(* Logix 5000 AddOnInstructionDefinition export Banner_TLF100_Param_v4; software revision 33.00 *)

TYPE Banner_IOL_Port_v4 :   // UDT that has all of the data items necessary to communicate with a specific Port on a IO-Link Master
STRUCT
   Port_Controlled : INT;   // Each bit represents a port on an IO-Link Master. Set to 1 to tell AOI to control that port.
   Port_Activate : INT;   // Each bit represents a port on an IO-Link Master. When ON that port will process any commands in queue.
   Port_Read : INT;   // Each bit represents a port on an IO-Link Master. Used to determine when device AOI has requested a Read command.
   Port_Write : INT;   // Each bit represents a port on an IO-Link Master. Used to determine when device AOI has requested a Write command.
   Port_RW_Complete : INT;   // Each bit represents a port on an IO-Link Master. Tells device AOI that Read or Write request has been completed.
   Port_Device_Read : INT;
   Data_Transfer : SINT[190];   // Array to transfer data from IO-Master to device AOIs.
END_STRUCT
END_TYPE

TYPE Banner_TLF100_General_Level_Config_v4 :
STRUCT
   BG_Color : SINT;   // Background Color. 0 = Green, 1 = Red, 2 = Orange, 3 = Amber, 4 = Yellow, 5 = Lime Green, 6 = Spring Green, 7 = Cyan, 8 = Sky Blue, 9 = Blue, 10 = Violet, 11 = Magenta, 12 = Rose, 13 = White, 14 = Custom, 15 = Custom 2.
   BG_Intensity : SINT;   // 0 = High, 1 = Low, 2 = Medium, 3 = Off, 4 = Custom
   Dominance : SINT;   // 0 = Non-Dominant, 1 = Dominant
   Sub_Segment_Style : SINT;   // 0 = Solid, 1 = Analog
   Filtering : SINT;   // 0 = None, 1 = Low, 2 = Medium, 3 = High
   Hysteresis : SINT;   // 0 = None, 1 = Low, 2 = Medium, 3 = High
   Full_Scale_Value : INT;   // Default value is 100
END_STRUCT
END_TYPE

TYPE Banner_TLF100_General_Seg_Config_v4 :
STRUCT
   Segment_Mode : INT;   // 0 = Manual Segment Config, 1 = 1 Segment, 2 = 2 Segments, 3 = 3 Segments, 4 = 4 Segments
   Background_Color : INT;   // 0 = Green, 1 = Red, 2 = Orange, 3 = Amber, 4 = Yellow, 5 = Lime Green, 6 = Spring Green, 7 = Cyan, 8 = Sky Blue, 9 = Blue, 10 = Violet, 11 = Magenta, 12 = Rose, 13 = White, 14 = Custom, 15 = Custom 2
   Background_Intensity : SINT;   // 0 = High, 1 = Low, 2 = Medium, 3 = Off, 4 = Custom
   Animation_Synchro : SINT;   // 0 = Animation Sync Disabled, 1 = Animation Sync Enabled
END_STRUCT
END_TYPE

TYPE Banner_TLF100_Level_Base_Config_v4 :
STRUCT
   Animation : INT;   // 0 = Off, 1 = Steady, 2 = Flash, 3 = Two Color Flash, 4 = Two Color Shift, 5 = Scroll, 6 = Center Scroll, 7 = Bounce, 8 = Center Bounce, 9 = Intensity Sweep, 10 = Two Color Sweep, 11 = Spectrum, 12 = Single End Steady, 13 = Daylight White, 14 = Custom 1, 15 = Custom 2
   Color_1 : INT;   // 0 = Green, 1 = Red, 2 = Orange, 3 = Amber, 4 = Yellow, 5 = Lime Green, 6 = Spring Green, 7 = Cyan, 8 = Sky Blue, 9 = Blue, 10 = Violet, 11 = Magenta, 12 = Rose, 13 = White, 14 = Custom, 15 = Custom 2
   Color_1_Intensity : SINT;   // 0 = High, 1 = Low, 2 = Medium, 3 = Off, 4 = Custom
   Speed : SINT;   // 0 = Medium, 1 = Fast, 2 = Slow, 3 = Custom Flash Rate
   Pulse_Pattern : SINT;   // 0 = Normal, 1 = Strobe, 2 = Three Pulse, 3 = SOS, 4 = Random
   Color_2 : INT;   // 0 = Green, 1 = Red, 2 = Orange, 3 = Amber, 4 = Yellow, 5 = Lime Green, 6 = Spring Green, 7 = Cyan, 8 = Sky Blue, 9 = Blue, 10 = Violet, 11 = Magenta, 12 = Rose, 13 = White, 14 = Custom, 15 = Custom 2
   Color_2_Intensity : INT;   // 0 = High, 1 = Low, 2 = Medium, 3 = Off, 4 = Custom
   Scroll_Bounce_Style : SINT;   // 0 = Solid, 1 = Tail, 2 = Ripple
   Percent_Width_of_Color_1 : SINT;   // 0 to 100. The size of the scrolling segement
   Direction : SINT;   // 0 = Up, 1 = Down
   Audible : SINT;   // 0 = Pulse, 1 = Wobble, 2 = Strobe, 4 = Whoop, 5 = Stacatto, 6 = Siren, 8 = Continuous 1, 9 = Continuous 2, 16 = Jingle, 17 = Melody 1, 18 = Melody 2, 19 = Melody 3, 20 = Custom
   Audible_Volume : SINT;   // 0 = Off, 1 = Low, 2 = Medium, 3 = High
END_STRUCT
END_TYPE

TYPE Banner_TLF100_RD_v4 :   // UDT that stores the Read Data for a TLF100 Pro.
STRUCT
   Master_Cycle_Time : INT;
   Min_Cycle_Time : INT;
   M_Sequence_Capability : INT;
   IO_Link_Version_ID : INT;
   Process_Data_Input_Length : INT;
   Process_Data_Output_Length : INT;
   Combined_Vendor_ID : DINT;   // IO-Link Vendor ID
   Vendor_ID1 : INT;
   Vendor_ID2 : INT;
   Combined_Device_ID : DINT;   // IO-Link Device ID
   Device_ID1 : INT;
   Device_ID2 : INT;
   Device_ID3 : INT;
   Serial_Number : STRING;
END_STRUCT
END_TYPE

TYPE Banner_TLF100_SegConfig_v4 :   // Basic parameters for a TLF100 segment.
STRUCT
   Animation : SINT;   // 0 = Off, 1 = Steady, 2 = Flash, 3 = Two Color, 4 = Half/Half, 5 = Half/Half Rotate, 6 = Chase, 7 = Intesnity Sweep
   Color_1 : INT;   // 0 = Green, 1 = Red, 2 = Orange, 3 = Amber, 4 = Yellow, 5 = Lime Green, 6 = Spring Green, 7 = Cyan, 8 = Sky Blue, 9 = Blue, 10 = Violet, 11 = Magenta, 12 = Rose, 13 = White, 14 = Custom, 15 = Custom 2
   Color_1_Intensity : SINT;   // 0 = High, 1 = Low, 2 = Medium, 3 = Off, 4 = Custom
   Speed : SINT;   // 0 = Medium, 1 = Fast, 2 = Slow, 3 = Custom
   Pulse_Pattern : SINT;   // 0 = Normal, 1 = Strobe, 2 = Three Pulse, 3 = SOS, 4 = Random
   Color_2 : SINT;   // 0 = Green, 1 = Red, 2 = Orange, 3 = Amber, 4 = Yellow, 5 = Lime Green, 6 = Spring Green, 7 = Cyan, 8 = Sky Blue, 9 = Blue, 10 = Violet, 11 = Magenta, 12 = Rose, 13 = White, 14 = Custom, 15 = Custom 2
   Color_2_Intensity : SINT;   // 0 = High, 1 = Low, 2 = Medium, 3 = Off, 4 = Custom
   Scroll_Bounce : SINT;   // 0 = Solid, 1 = Tail, 2 = Ripple
   Percent_Width_of_C1 : SINT;   // 1 to 100 percent
   Direction : SINT;   // 0 = Up, 1 = Down
END_STRUCT
END_TYPE

TYPE Banner_TLF100_Threshold_Config_v4 :
STRUCT
   Threshold_Enable : SINT;   // 0 = Threshold Disabled, 1 = Threshold Enabled
   Threshold_Value_Percent : SINT;   // 0 to 100 percent.
   Threshold_Comparison : SINT;   // 0 = Less than or equal to, 1 = Greater than or equal to
   Threshold_Override : SINT;   // 0 = Override not enabled, 1 = Override Enabled
   Animation : INT;   // 0 = Off, 1 = Steady, 2 = Flash, 3 = Two Color Flash, 4 = Two Color Shift, 5 = Scroll, 6 = Center Scroll, 7 = Bounce, 8 = Center Bounce, 9 = Intensity Sweep, 10 = Two Color Sweep, 11 = Spectrum, 12 = Single End Steady, 13 = Single End Flash
   Color_1 : INT;   // 0 = Green, 1 = Red, 2 = Orange, 3 = Amber, 4 = Yellow, 5 = Lime Green, 6 = Spring Green, 7 = Cyan, 8 = Sky Blue, 9 = Blue, 10 = Violet, 11 = Magenta, 12 = Rose, 13 = White, 14 = Custom, 15 = Custom 2
   Color_1_Intensity : SINT;   // 0 = High, 1 = Low, 2 = Medium, 3 = Off, 4 = Custom
   Speed : SINT;   // 0 = Medium, 1 = Fast, 2 = Slow, 3 = Custom Flash Rate
   Pulse_Pattern : SINT;   // 0 = Normal, 1 = Strobe, 2 = Three Pulse, 3 = SOS, 4 = Random
   Color_2 : INT;   // 0 = Green, 1 = Red, 2 = Orange, 3 = Amber, 4 = Yellow, 5 = Lime Green, 6 = Spring Green, 7 = Cyan, 8 = Sky Blue, 9 = Blue, 10 = Violet, 11 = Magenta, 12 = Rose, 13 = White, 14 = Custom, 15 = Custom 2
   Color_2_Intensity : SINT;   // 0 = High, 1 = Low, 2 = Medium, 3 = Off, 4 = Custom
   Scroll_Bounce_Style : SINT;   // 0 = Solid, 1 = Tail, 2 = Ripple
   Percent_Width_of_Color_1 : SINT;   // 0 to 100
   Direction : SINT;   // 0 = Up, 1 = Down
   Audible_Type : SINT;   // 0 = Pulse, 1 = Wobble, 2 = Strobe, 4 = Whoop, 5 = Stacatto, 6 = Siren, 8 = Continuous 1, 9 = Continuous 2, 12 = Sync, 16 = Jingle, 17 = Melody 1, 18 = Melody 2, 19 = Melody 3, 20 = Custom
   Audible_Volume : SINT;   // 0 = Off, 1 = Low, 2 = Medium, 3 = High
END_STRUCT
END_TYPE

TYPE Banner_TLF100_v4 :   // All of the parameters for a TLF100.
STRUCT
   Initial_Global_Read : BOOL;   // Determines if all of the IO-Link data has been read into the PLC yet
   Command : INT;   // Value placed in here will activate a read or write to a specifc IO-Link Index
   Read : Banner_TLF100_RD_v4;   // Read Only Data
   Write : Banner_TLF100_WD_v4;   // Write Data
   Archive : Banner_TLF100_WD_v4;   // Archive of the Write Data
   Reset : BOOL;   // Resets AOI. This will force a complete parameter read of the sensor.
END_STRUCT
END_TYPE

TYPE Banner_TLF100_WD_v4 :   // UDT that stores the Write Data for a TLF100.
STRUCT
   System_Command : INT;   // See IODD file for list of commands that can be activated via the System Command interface
   Parameter_Access_Lock : SINT;   // Write access to all parameters is prohibited while value is 1. Only this parameter can be adjusted when value is 1.
   Data_Storage_Lock : SINT;   // Automatic data storage is disabled when this value is equal to 1. Read access is not affected.
   Local_Parameterization_Lock : SINT;   // Parameterization via local control elements on device is disabled.
   Local_User_Interface_Lock : SINT;   // Operation of local user interface is disabled.
   Operating_Mode_Selection : SINT;   // 0 = Segment Mode, 1 = Run Mode, 2= Level Mode, 3 = Adv Seg Mode, 4 = Demo Mode
   General_Segment_Config : Banner_TLF100_General_Seg_Config_v4;
   Segment_Config : Banner_TLF100_SegConfig_v4[5];
   General_Level_Config : Banner_TLF100_General_Level_Config_v4;
   Level_Base_Config : Banner_TLF100_Level_Base_Config_v4;
   Level_Threshold_Config : Banner_TLF100_Threshold_Config_v4[5];
   Custom_1_Red : INT;   // 0 to 255. Value of the Red portion of the RGB color value for Custom 1
   Custom_1_Green : INT;   // 0 to 255. Value of the Green portion of the RGB color value for Custom 1.
   Custom_1_Blue : INT;   // 0 to 255. Value of the Blue portion of the RGB color value for Custom 1.
   Custom_2_Red : INT;   // 0 to 255. Value of the Red portion of the RGB color value for Custom 2.
   Custom_2_Green : INT;   // 0 to 255. Value of the Green portion of the RGB color value for Custom 2.
   Custom_2_Blue : INT;   // 0 to 255. Value of the Blue portion of the RGB color value for Custom 2.
   Orientation : SINT;   // 0 = Standard, 1 = Inverted
   Custom_Intensity : SINT;   // 0 to 100
   Custom_Frequency : INT;   // 0 to 255
   Audible : SINT;   // 0 = Pulse, 1 = Wobble, 2 = Strobe, 4 = Whoop, 5 = Stacatto, 6 = Siren, 8 = Continuous 1, 9 = Continuous 2, 16 = Jingle, 17 = Melody 1, 18 = Melody 2, 19 = Melody 3, 20 = Custom
   Audible_Volume : SINT;   // 0 = Off, 1 = Low, 2 = Medium, 3 = High
   Custom_Type : SINT;   // 0 = Beep, 1 = Sweep, 2 = Tone
   Custom_Sweep_Type : SINT;   // 0 = Up, 1 = Down, 2 = Up Down, 3 = Down Up
   Custom_Freq_1 : SINT;   // 0 = Off, 1 = Low, 2 = Standard, 3 = High
   Custom_Freq_2 : SINT;   // 0 = Off, 1 = Low, 2 = Standard, 3 = High
END_STRUCT
END_TYPE

ADD_ON_INSTRUCTION Banner_TLF100_Param_v4   (* revision 4.1, vendor Banner Engineering *)
// AOI to read and write parameter data to an IO-Link TLF100.
VAR_IN_OUT
   TLF100 : Banner_TLF100_v4; {required}
   Port_Data : Banner_IOL_Port_v4; {required}
END_VAR
VAR_INPUT
   Port : INT; {required}   // Port Number that device is plugged into.
END_VAR
VAR
   Local_Control : DINT; {access None}
   Global_Read_Command_Value : INT; {access None}
   Global_Write_Command_Value : INT; {access None}
   Command_Being_Processed : BOOL; {access None}
   Update_Archive : BOOL; {access None}
   Index_Write_Inprocess : DINT; {access None}
   Index_Write_Control : DINT; {access None}
   Inprocess_Index : DINT; {access None}
   Index_R : DINT; {access None}
   BS_Index : DINT; {access None}
   Index_W : DINT; {access None}
   W_Index : DINT; {access None}
   Index_Segment_Read : DINT; {access None}
   GT_Index2 : DINT; {access None}
   GT_Index1 : DINT; {access None}
   LT_Index2 : DINT; {access None}
   LT_Index1 : DINT; {access None}
END_VAR

ROUTINE Logic   (* ladder *)
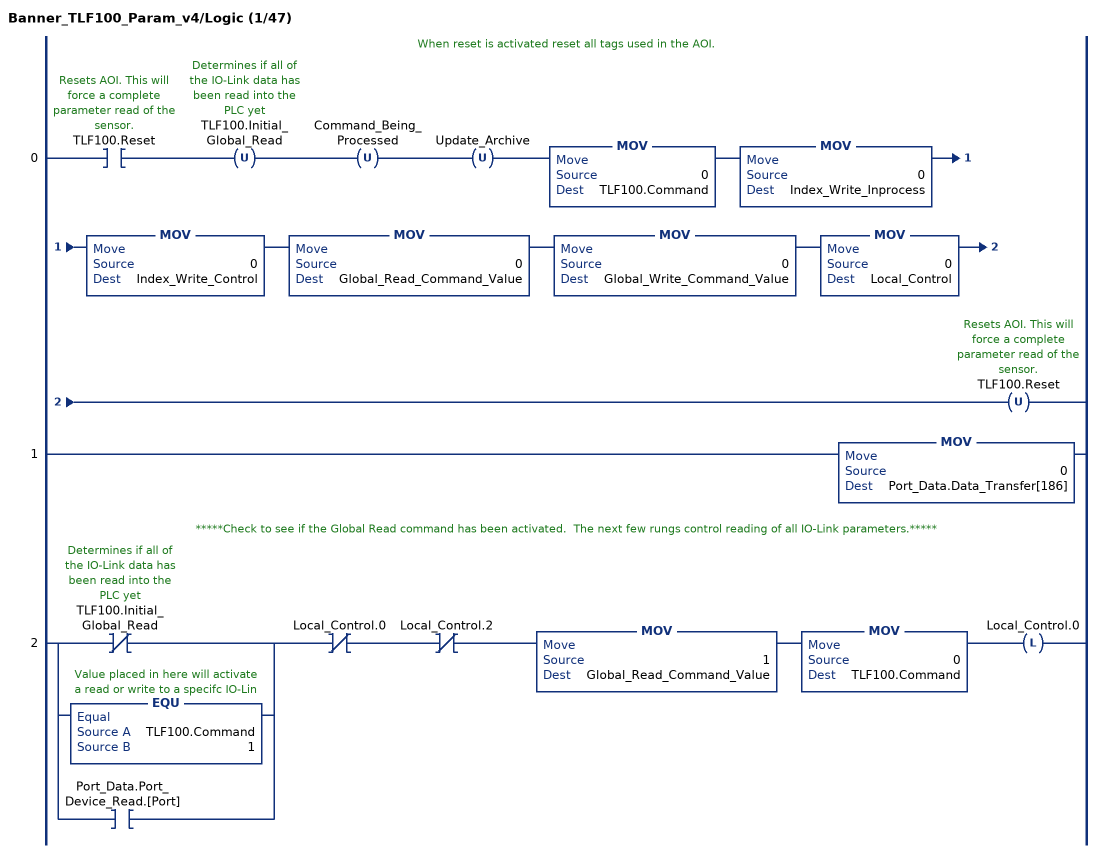
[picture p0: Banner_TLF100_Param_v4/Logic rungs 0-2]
   // When reset is activated reset all tags used in the AOI.
   0: XIC(TLF100.Reset)OTU(TLF100.Initial_Global_Read)OTU(Command_Being_Processed)OTU(Update_Archive)MOV(0,TLF100.Command)MOV(0,Index_Write_Inprocess)MOV(0,Index_Write_Control)MOV(0,Global_Read_Command_Value)MOV(0,Global_Write_Command_Value)MOV(0,Local_Control)OTU(TLF100.Reset);
   1: MOV(0,Port_Data.Data_Transfer[186]);
   // *****Check to see if the Global Read command has been activated.  The next few rungs control reading of all IO-Link parameters.*****
   2: [XIO(TLF100.Initial_Global_Read) ,EQU(TLF100.Command,1) ,XIC(Port_Data.Port_Device_Read.[Port]) ]XIO(Local_Control.0)XIO(Local_Control.2)MOV(1,Global_Read_Command_Value)MOV(0,TLF100.Command)OTL(Local_Control.0);
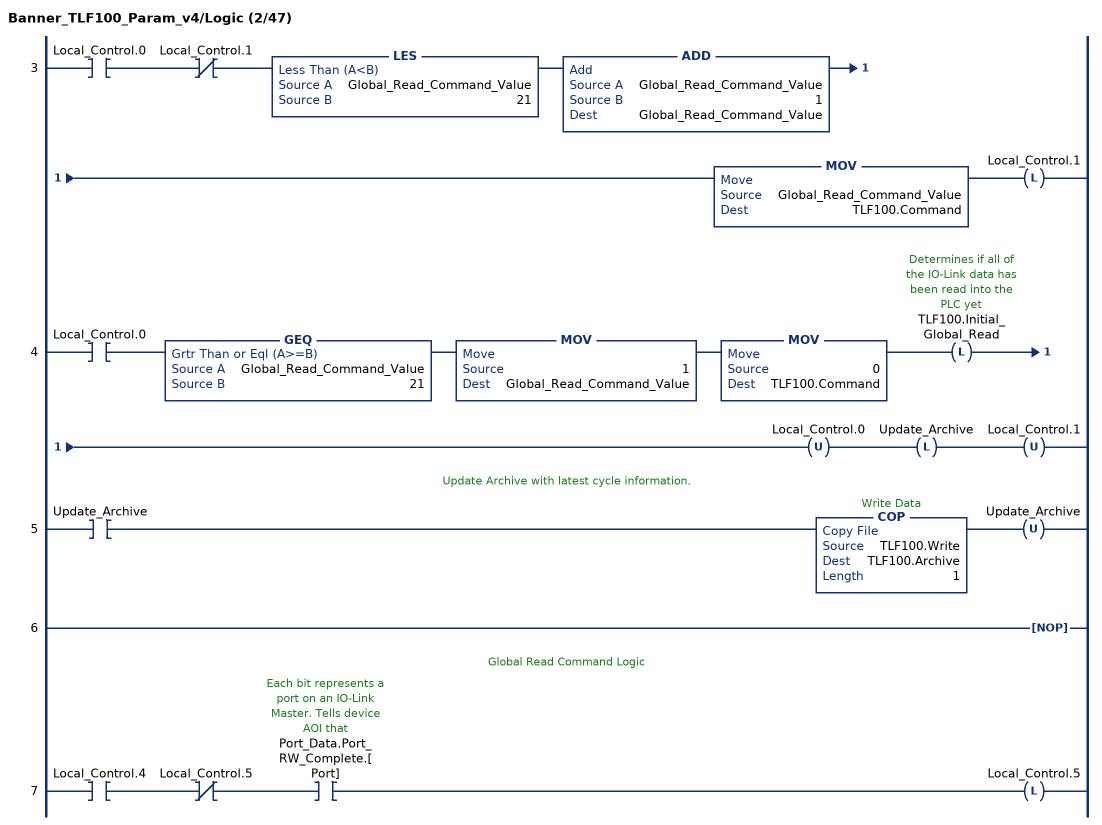
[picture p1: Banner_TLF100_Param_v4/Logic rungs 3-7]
   3: XIC(Local_Control.0)XIO(Local_Control.1)LES(Global_Read_Command_Value,21)ADD(Global_Read_Command_Value,1,Global_Read_Command_Value)MOV(Global_Read_Command_Value,TLF100.Command)OTL(Local_Control.1);
   4: XIC(Local_Control.0)GEQ(Global_Read_Command_Value,21)MOV(1,Global_Read_Command_Value)MOV(0,TLF100.Command)OTL(TLF100.Initial_Global_Read)OTU(Local_Control.0)OTL(Update_Archive)OTU(Local_Control.1);
   // Update Archive with latest cycle information.
   5: XIC(Update_Archive)COP(TLF100.Write,TLF100.Archive,1)OTU(Update_Archive);
   6: NOP();
   // Global Read Command Logic
   7: XIC(Local_Control.4)XIO(Local_Control.5)XIC(Port_Data.Port_RW_Complete.[Port])OTL(Local_Control.5);
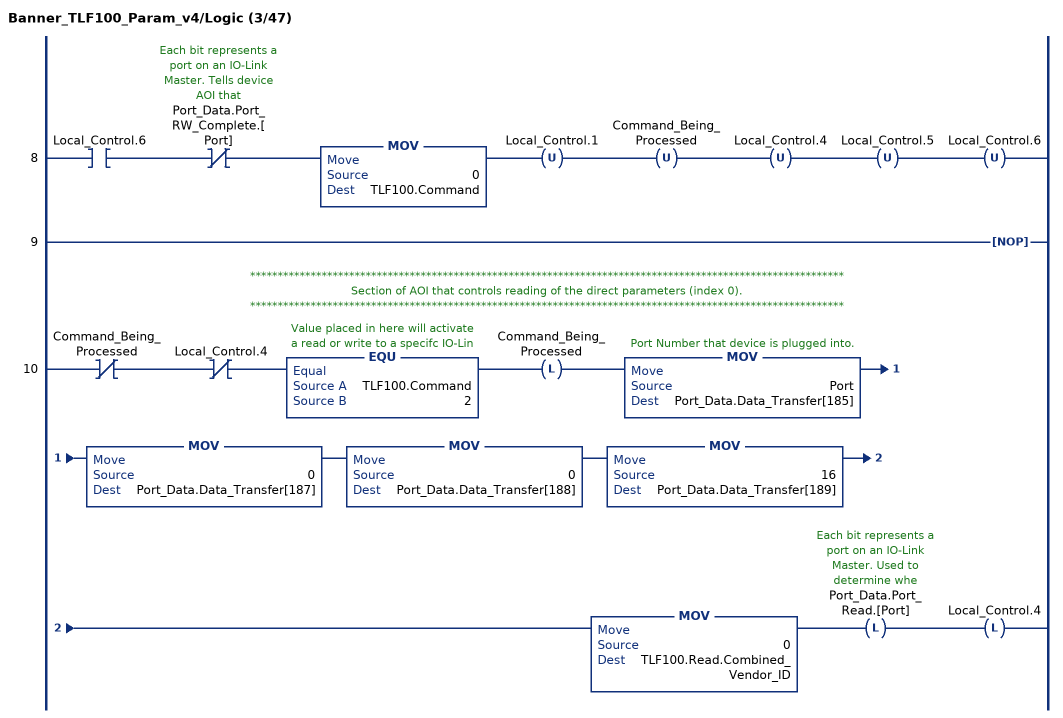
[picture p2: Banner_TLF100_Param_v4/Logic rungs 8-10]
   8: XIC(Local_Control.6)XIO(Port_Data.Port_RW_Complete.[Port])MOV(0,TLF100.Command)OTU(Local_Control.1)OTU(Command_Being_Processed)OTU(Local_Control.4)OTU(Local_Control.5)OTU(Local_Control.6);
   9: NOP();
   // ************************************************************************************************************
   // Section of AOI that controls reading of the direct parameters (index 0).
   // ************************************************************************************************************
   10: XIO(Command_Being_Processed)XIO(Local_Control.4)EQU(TLF100.Command,2)OTL(Command_Being_Processed)MOV(Port,Port_Data.Data_Transfer[185])MOV(0,Port_Data.Data_Transfer[187])MOV(0,Port_Data.Data_Transfer[188])MOV(16,Port_Data.Data_Transfer[189])MOV(0,TLF100.Read.Combined_Vendor_ID)OTL(Port_Data.Port_Read.[Port])OTL(Local_Control.4);
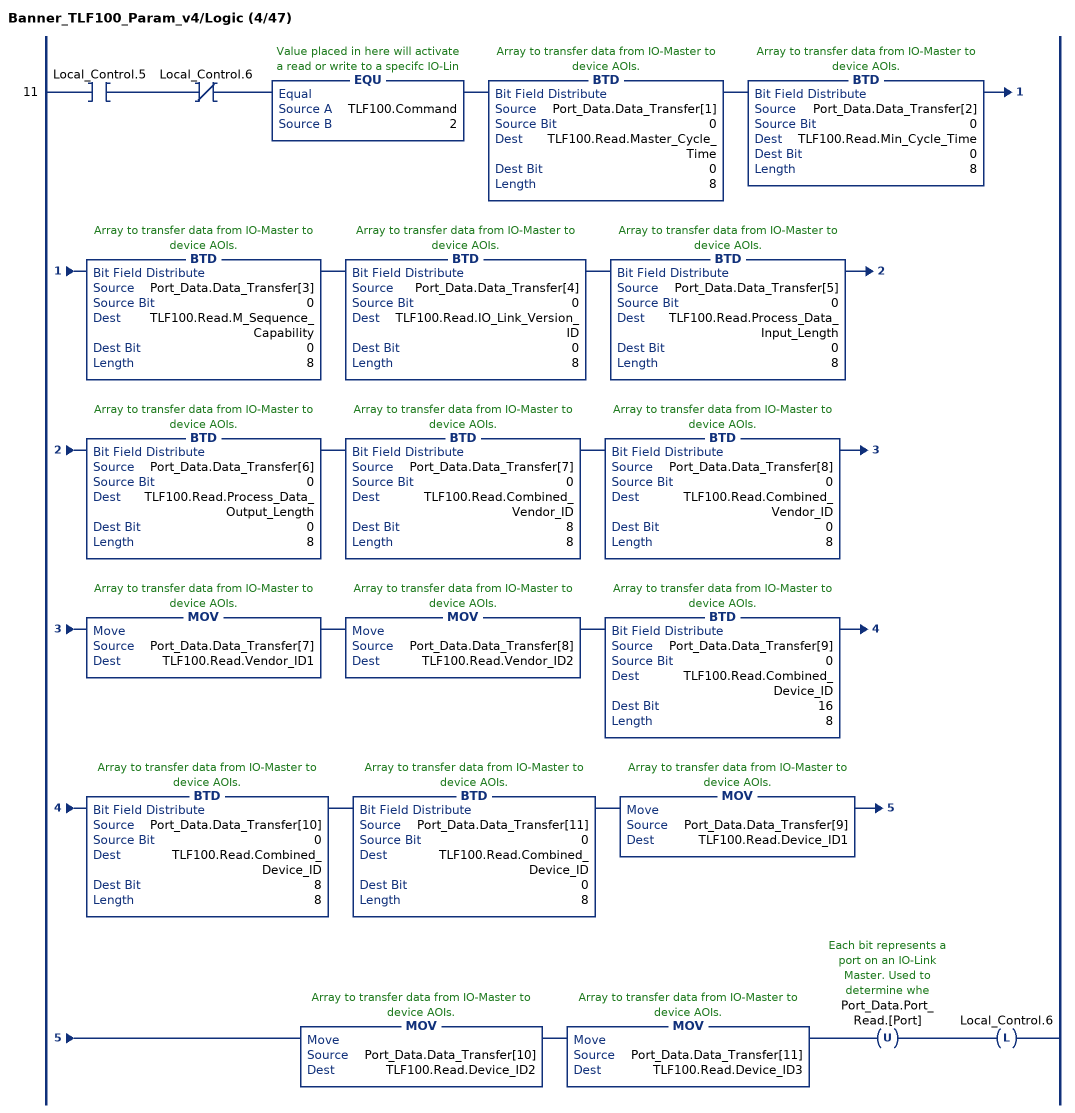
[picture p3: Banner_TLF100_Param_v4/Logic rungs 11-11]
   11: XIC(Local_Control.5)XIO(Local_Control.6)EQU(TLF100.Command,2)BTD(Port_Data.Data_Transfer[1],0,TLF100.Read.Master_Cycle_Time,0,8)BTD(Port_Data.Data_Transfer[2],0,TLF100.Read.Min_Cycle_Time,0,8)BTD(Port_Data.Data_Transfer[3],0,TLF100.Read.M_Sequence_Capability,0,8)BTD(Port_Data.Data_Transfer[4],0,TLF100.Read.IO_Link_Version_ID,0,8)BTD(Port_Data.Data_Transfer[5],0,TLF100.Read.Process_Data_Input_Length,0,8)BTD(Port_Data.Data_Transfer[6],0,TLF100.Read.Process_Data_Output_Length,0,8)BTD(Port_Data.Data_Transfer[7],0,TLF100.Read.Combined_Vendor_ID,8,8)BTD(Port_Data.Data_Transfer[8],0,TLF100.Read.Combined_Vendor_ID,0,8)MOV(Port_Data.Data_Transfer[7],TLF100.Read.Vendor_ID1)MOV(Port_Data.Data_Transfer[8],TLF100.Read.Vendor_ID2)BTD(Port_Data.Data_Transfer[9],0,TLF100.Read.Combined_Device_ID,16,8)BTD(Port_Data.Data_Transfer[10],0,TLF100.Read.Combined_Device_ID,8,8)BTD(Port_Data.Data_Transfer[11],0,TLF100.Read.Combined_Device_ID,0,8)MOV(Port_Data.Data_Transfer[9],TLF100.Read.Device_ID1)MOV(Port_Data.Data_Transfer[10],TLF100.Read.Device_ID2)MOV(Port_Data.Data_Transfer[11],TLF100.Read.Device_ID3)OTU(Port_Data.Port_Read.[Port])OTL(Local_Control.6);
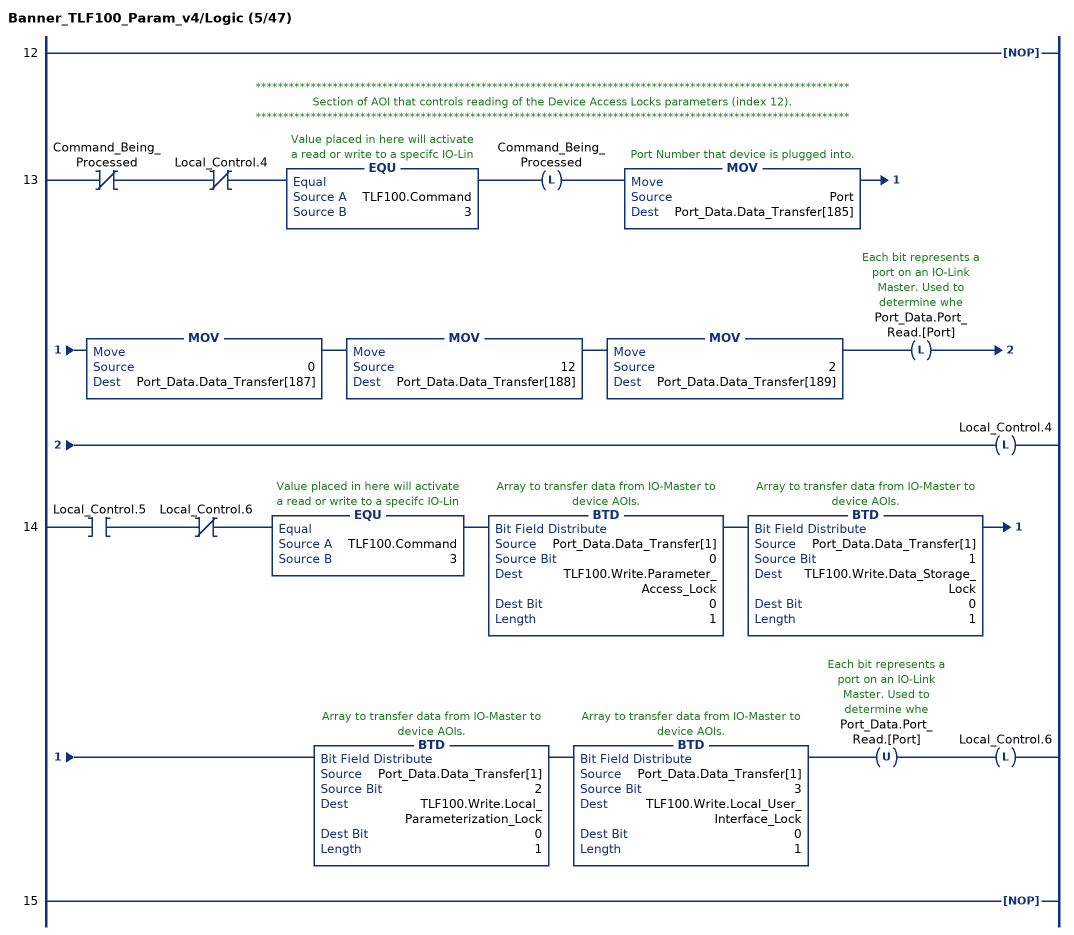
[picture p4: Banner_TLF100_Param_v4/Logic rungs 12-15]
   12: NOP();
   // ************************************************************************************************************
   // Section of AOI that controls reading of the Device Access Locks parameters (index 12).
   // ************************************************************************************************************
   13: XIO(Command_Being_Processed)XIO(Local_Control.4)EQU(TLF100.Command,3)OTL(Command_Being_Processed)MOV(Port,Port_Data.Data_Transfer[185])MOV(0,Port_Data.Data_Transfer[187])MOV(12,Port_Data.Data_Transfer[188])MOV(2,Port_Data.Data_Transfer[189])OTL(Port_Data.Port_Read.[Port])OTL(Local_Control.4);
   14: XIC(Local_Control.5)XIO(Local_Control.6)EQU(TLF100.Command,3)BTD(Port_Data.Data_Transfer[1],0,TLF100.Write.Parameter_Access_Lock,0,1)BTD(Port_Data.Data_Transfer[1],1,TLF100.Write.Data_Storage_Lock,0,1)BTD(Port_Data.Data_Transfer[1],2,TLF100.Write.Local_Parameterization_Lock,0,1)BTD(Port_Data.Data_Transfer[1],3,TLF100.Write.Local_User_Interface_Lock,0,1)OTU(Port_Data.Port_Read.[Port])OTL(Local_Control.6);
   15: NOP();
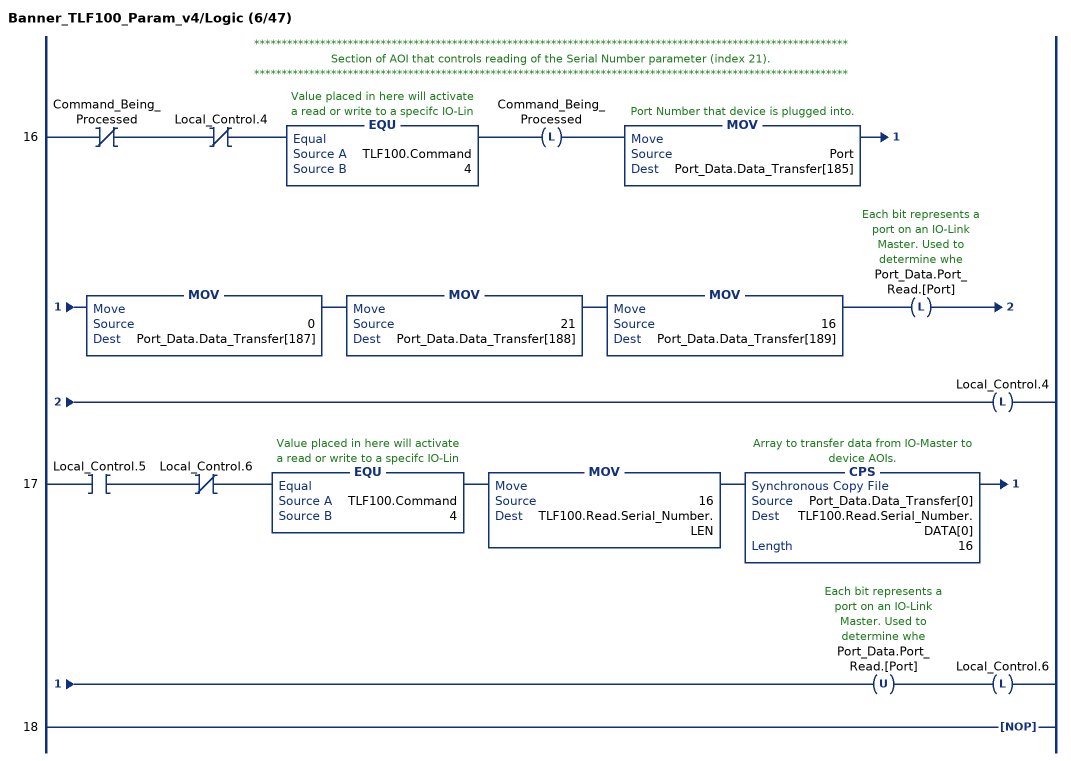
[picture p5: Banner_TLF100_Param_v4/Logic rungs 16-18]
   // ************************************************************************************************************
   // Section of AOI that controls reading of the Serial Number parameter (index 21).
   // ************************************************************************************************************
   16: XIO(Command_Being_Processed)XIO(Local_Control.4)EQU(TLF100.Command,4)OTL(Command_Being_Processed)MOV(Port,Port_Data.Data_Transfer[185])MOV(0,Port_Data.Data_Transfer[187])MOV(21,Port_Data.Data_Transfer[188])MOV(16,Port_Data.Data_Transfer[189])OTL(Port_Data.Port_Read.[Port])OTL(Local_Control.4);
   17: XIC(Local_Control.5)XIO(Local_Control.6)EQU(TLF100.Command,4)MOV(16,TLF100.Read.Serial_Number.LEN)CPS(Port_Data.Data_Transfer[0],TLF100.Read.Serial_Number.DATA[0],16)OTU(Port_Data.Port_Read.[Port])OTL(Local_Control.6);
   18: NOP();
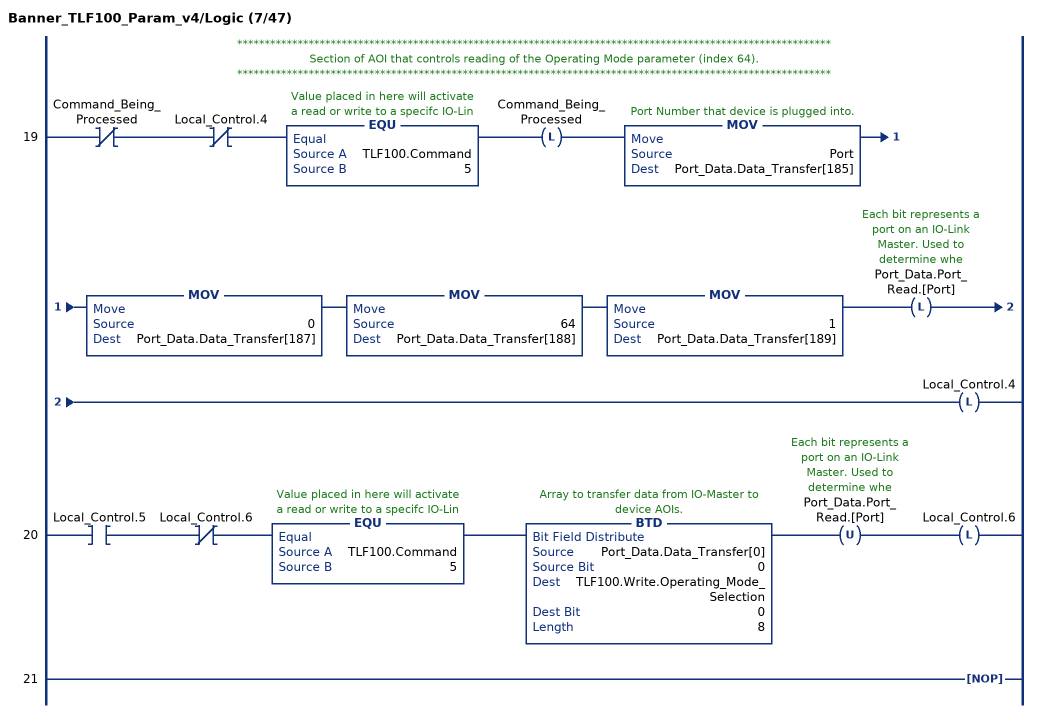
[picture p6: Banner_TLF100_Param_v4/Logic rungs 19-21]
   // ************************************************************************************************************
   // Section of AOI that controls reading of the Operating Mode parameter (index 64).
   // ************************************************************************************************************
   19: XIO(Command_Being_Processed)XIO(Local_Control.4)EQU(TLF100.Command,5)OTL(Command_Being_Processed)MOV(Port,Port_Data.Data_Transfer[185])MOV(0,Port_Data.Data_Transfer[187])MOV(64,Port_Data.Data_Transfer[188])MOV(1,Port_Data.Data_Transfer[189])OTL(Port_Data.Port_Read.[Port])OTL(Local_Control.4);
   20: XIC(Local_Control.5)XIO(Local_Control.6)EQU(TLF100.Command,5)BTD(Port_Data.Data_Transfer[0],0,TLF100.Write.Operating_Mode_Selection,0,8)OTU(Port_Data.Port_Read.[Port])OTL(Local_Control.6);
   21: NOP();
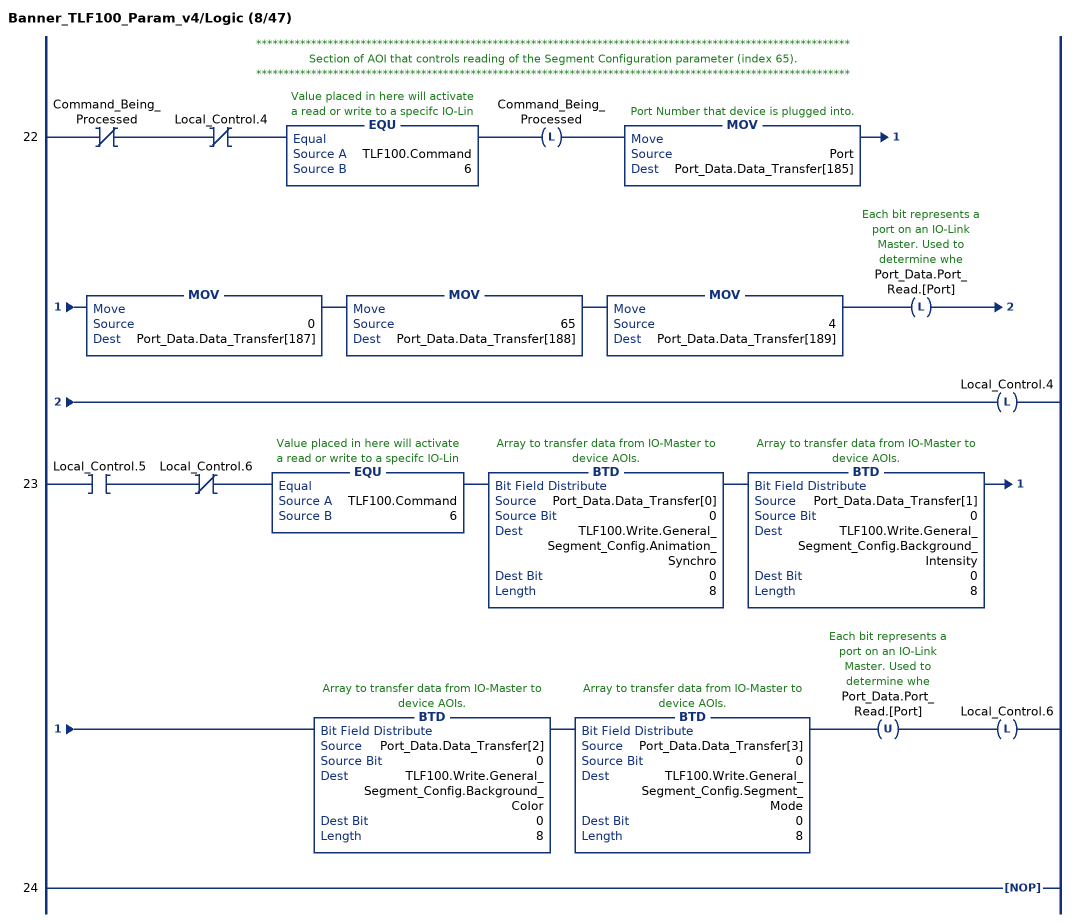
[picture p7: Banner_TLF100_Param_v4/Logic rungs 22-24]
   // ************************************************************************************************************
   // Section of AOI that controls reading of the Segment Configuration parameter (index 65).
   // ************************************************************************************************************
   22: XIO(Command_Being_Processed)XIO(Local_Control.4)EQU(TLF100.Command,6)OTL(Command_Being_Processed)MOV(Port,Port_Data.Data_Transfer[185])MOV(0,Port_Data.Data_Transfer[187])MOV(65,Port_Data.Data_Transfer[188])MOV(4,Port_Data.Data_Transfer[189])OTL(Port_Data.Port_Read.[Port])OTL(Local_Control.4);
   23: XIC(Local_Control.5)XIO(Local_Control.6)EQU(TLF100.Command,6)BTD(Port_Data.Data_Transfer[0],0,TLF100.Write.General_Segment_Config.Animation_Synchro,0,8)BTD(Port_Data.Data_Transfer[1],0,TLF100.Write.General_Segment_Config.Background_Intensity,0,8)BTD(Port_Data.Data_Transfer[2],0,TLF100.Write.General_Segment_Config.Background_Color,0,8)BTD(Port_Data.Data_Transfer[3],0,TLF100.Write.General_Segment_Config.Segment_Mode,0,8)OTU(Port_Data.Port_Read.[Port])OTL(Local_Control.6);
   24: NOP();
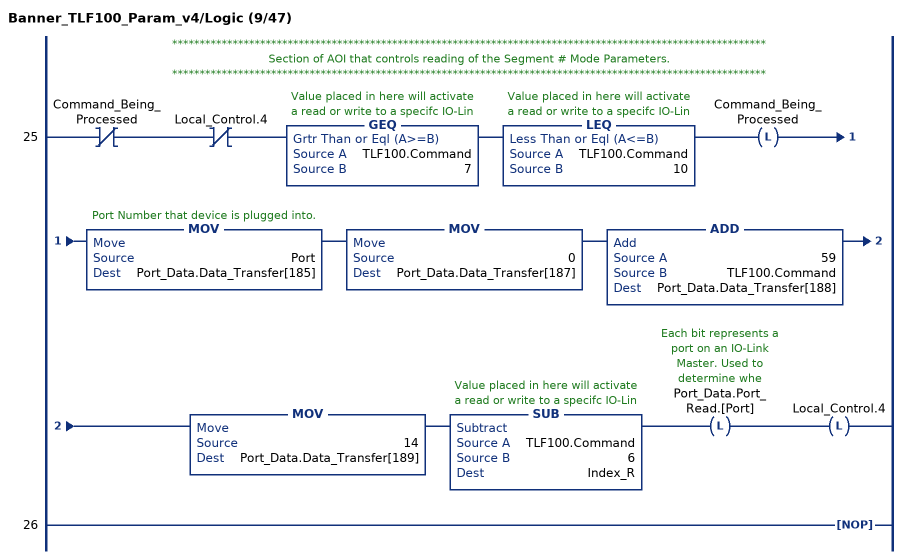
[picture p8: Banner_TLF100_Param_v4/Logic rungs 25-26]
   // ************************************************************************************************************
   // Section of AOI that controls reading of the Segment # Mode Parameters.
   // ************************************************************************************************************
   25: XIO(Command_Being_Processed)XIO(Local_Control.4)GEQ(TLF100.Command,7)LEQ(TLF100.Command,10)OTL(Command_Being_Processed)MOV(Port,Port_Data.Data_Transfer[185])MOV(0,Port_Data.Data_Transfer[187])ADD(59,TLF100.Command,Port_Data.Data_Transfer[188])MOV(14,Port_Data.Data_Transfer[189])SUB(TLF100.Command,6,Index_R)OTL(Port_Data.Port_Read.[Port])OTL(Local_Control.4);
   26: NOP();
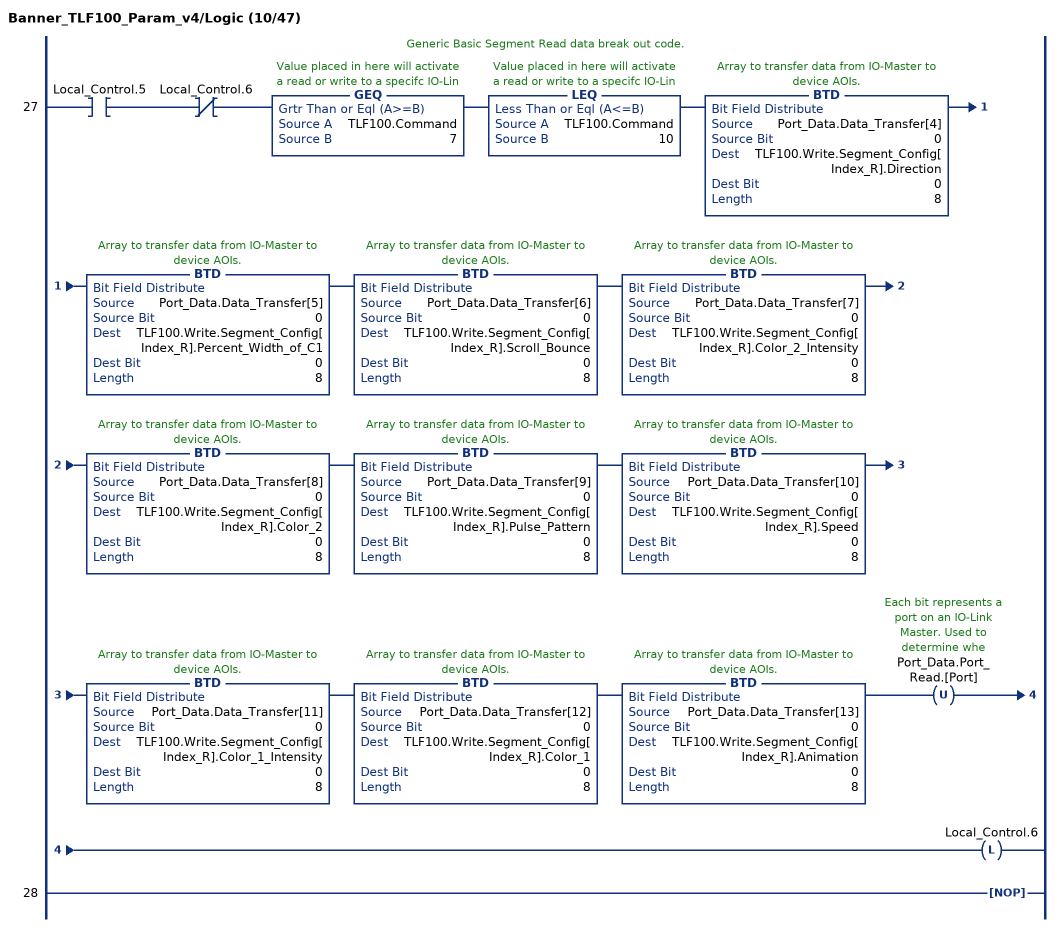
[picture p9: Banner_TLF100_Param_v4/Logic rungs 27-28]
   // Generic Basic Segment Read data break out code.
   27: XIC(Local_Control.5)XIO(Local_Control.6)GEQ(TLF100.Command,7)LEQ(TLF100.Command,10)BTD(Port_Data.Data_Transfer[4],0,TLF100.Write.Segment_Config[Index_R].Direction,0,8)BTD(Port_Data.Data_Transfer[5],0,TLF100.Write.Segment_Config[Index_R].Percent_Width_of_C1,0,8)BTD(Port_Data.Data_Transfer[6],0,TLF100.Write.Segment_Config[Index_R].Scroll_Bounce,0,8)BTD(Port_Data.Data_Transfer[7],0,TLF100.Write.Segment_Config[Index_R].Color_2_Intensity,0,8)BTD(Port_Data.Data_Transfer[8],0,TLF100.Write.Segment_Config[Index_R].Color_2,0,8)BTD(Port_Data.Data_Transfer[9],0,TLF100.Write.Segment_Config[Index_R].Pulse_Pattern,0,8)BTD(Port_Data.Data_Transfer[10],0,TLF100.Write.Segment_Config[Index_R].Speed,0,8)BTD(Port_Data.Data_Transfer[11],0,TLF100.Write.Segment_Config[Index_R].Color_1_Intensity,0,8)BTD(Port_Data.Data_Transfer[12],0,TLF100.Write.Segment_Config[Index_R].Color_1,0,8)BTD(Port_Data.Data_Transfer[13],0,TLF100.Write.Segment_Config[Index_R].Animation,0,8)OTU(Port_Data.Port_Read.[Port])OTL(Local_Control.6);
   28: NOP();
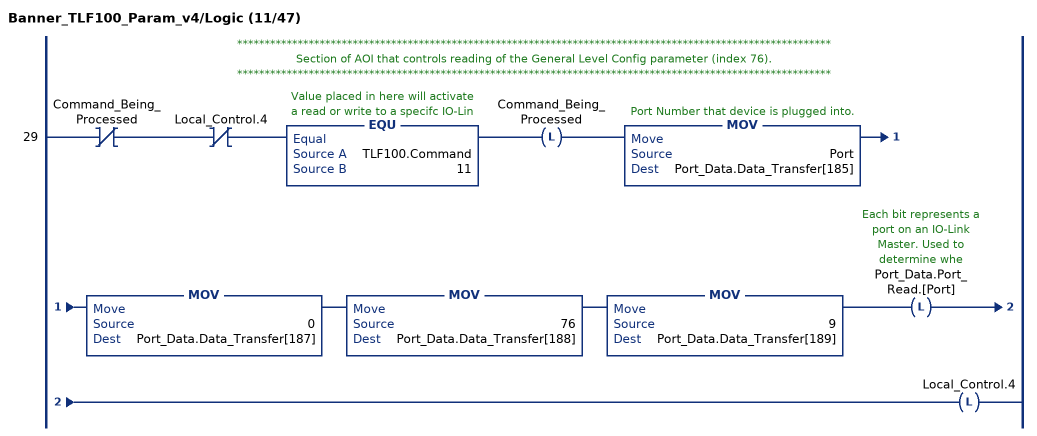
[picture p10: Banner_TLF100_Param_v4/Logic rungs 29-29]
   // ************************************************************************************************************
   // Section of AOI that controls reading of the General Level Config parameter (index 76).
   // ************************************************************************************************************
   29: XIO(Command_Being_Processed)XIO(Local_Control.4)EQU(TLF100.Command,11)OTL(Command_Being_Processed)MOV(Port,Port_Data.Data_Transfer[185])MOV(0,Port_Data.Data_Transfer[187])MOV(76,Port_Data.Data_Transfer[188])MOV(9,Port_Data.Data_Transfer[189])OTL(Port_Data.Port_Read.[Port])OTL(Local_Control.4);
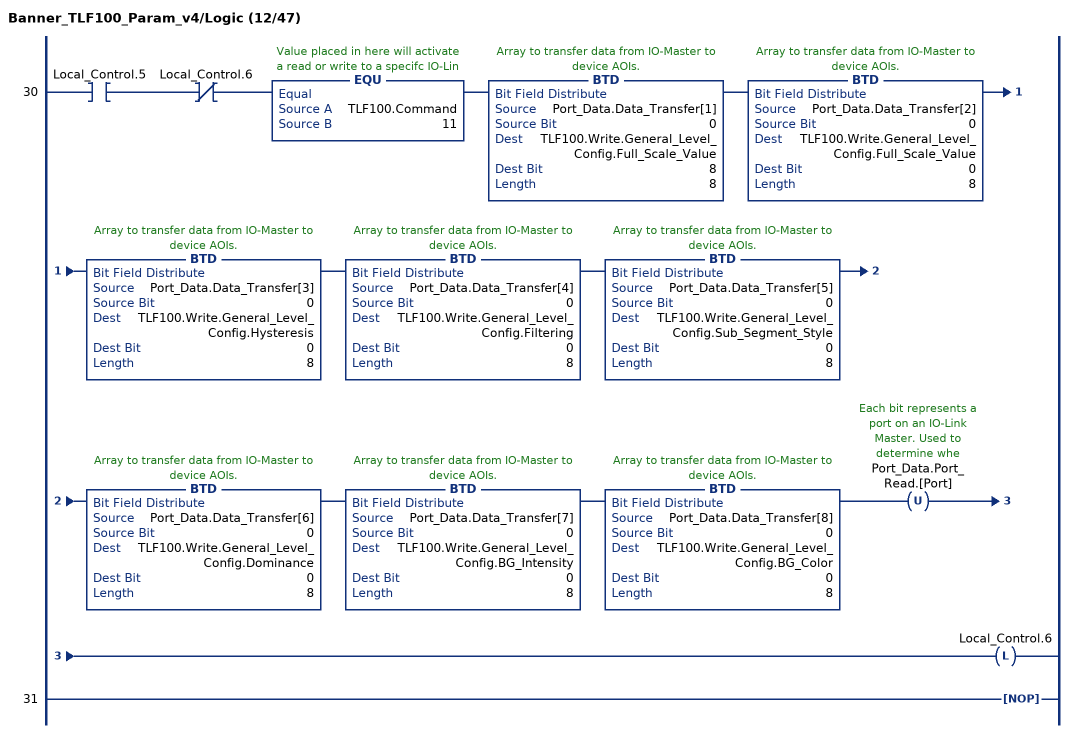
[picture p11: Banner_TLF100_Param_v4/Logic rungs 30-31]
   30: XIC(Local_Control.5)XIO(Local_Control.6)EQU(TLF100.Command,11)BTD(Port_Data.Data_Transfer[1],0,TLF100.Write.General_Level_Config.Full_Scale_Value,8,8)BTD(Port_Data.Data_Transfer[2],0,TLF100.Write.General_Level_Config.Full_Scale_Value,0,8)BTD(Port_Data.Data_Transfer[3],0,TLF100.Write.General_Level_Config.Hysteresis,0,8)BTD(Port_Data.Data_Transfer[4],0,TLF100.Write.General_Level_Config.Filtering,0,8)BTD(Port_Data.Data_Transfer[5],0,TLF100.Write.General_Level_Config.Sub_Segment_Style,0,8)BTD(Port_Data.Data_Transfer[6],0,TLF100.Write.General_Level_Config.Dominance,0,8)BTD(Port_Data.Data_Transfer[7],0,TLF100.Write.General_Level_Config.BG_Intensity,0,8)BTD(Port_Data.Data_Transfer[8],0,TLF100.Write.General_Level_Config.BG_Color,0,8)OTU(Port_Data.Port_Read.[Port])OTL(Local_Control.6);
   31: NOP();
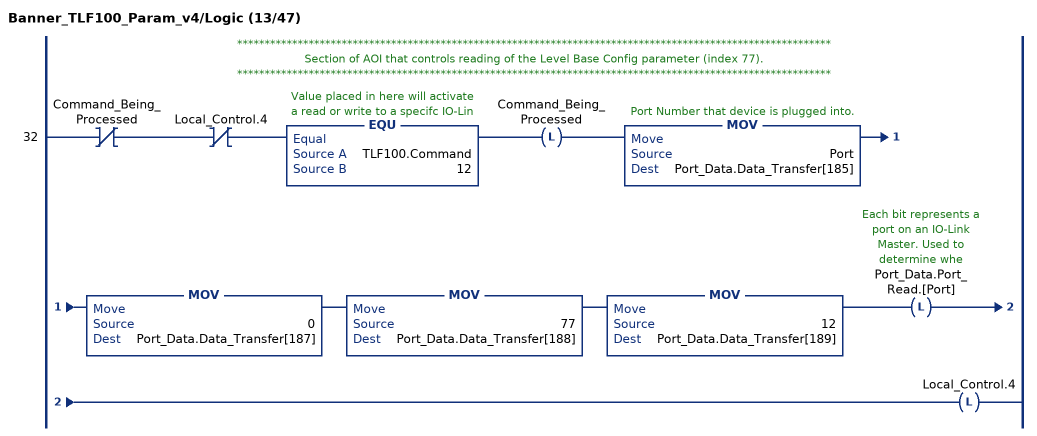
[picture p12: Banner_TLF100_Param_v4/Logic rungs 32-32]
   // ************************************************************************************************************
   // Section of AOI that controls reading of the Level Base Config parameter (index 77).
   // ************************************************************************************************************
   32: XIO(Command_Being_Processed)XIO(Local_Control.4)EQU(TLF100.Command,12)OTL(Command_Being_Processed)MOV(Port,Port_Data.Data_Transfer[185])MOV(0,Port_Data.Data_Transfer[187])MOV(77,Port_Data.Data_Transfer[188])MOV(12,Port_Data.Data_Transfer[189])OTL(Port_Data.Port_Read.[Port])OTL(Local_Control.4);
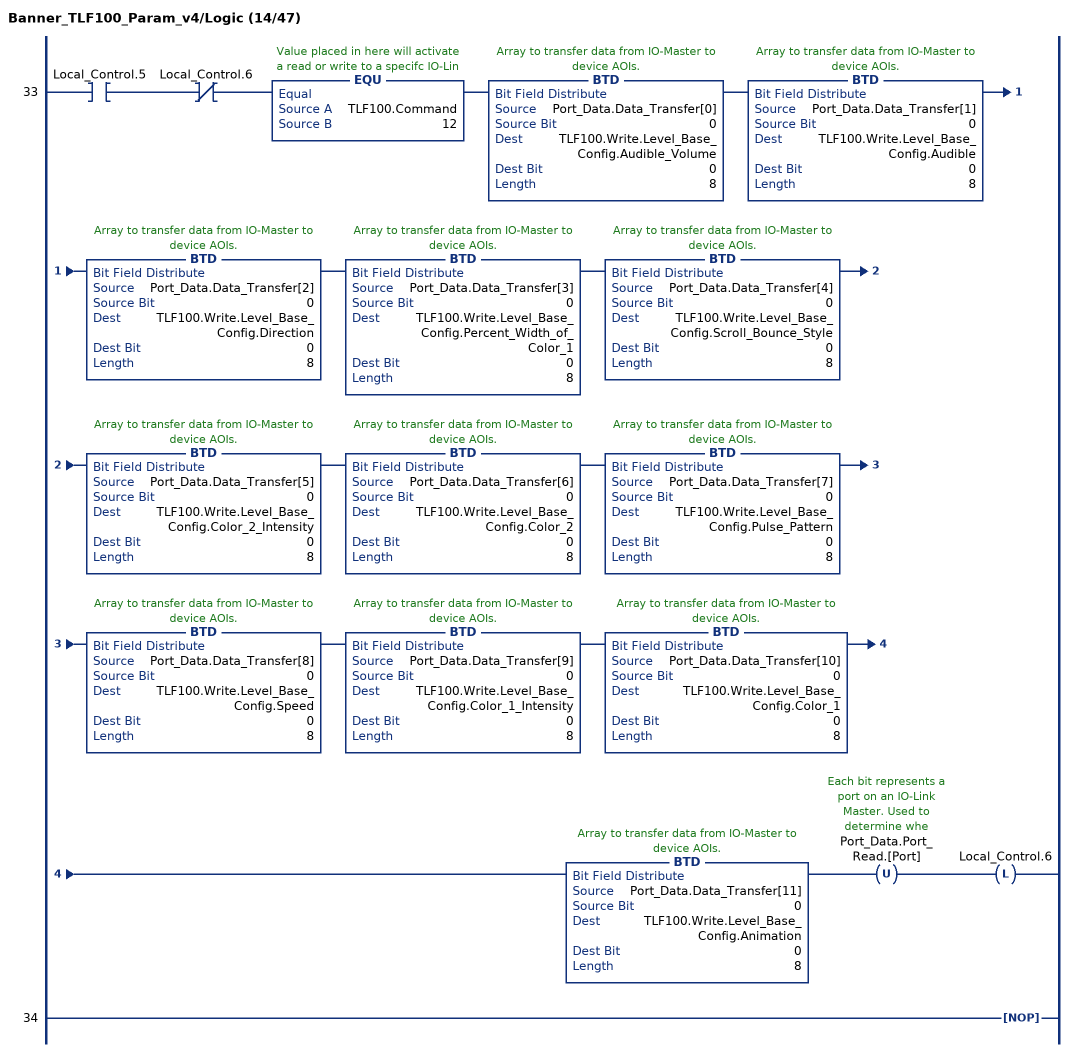
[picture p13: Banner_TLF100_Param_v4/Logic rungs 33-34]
   33: XIC(Local_Control.5)XIO(Local_Control.6)EQU(TLF100.Command,12)BTD(Port_Data.Data_Transfer[0],0,TLF100.Write.Level_Base_Config.Audible_Volume,0,8)BTD(Port_Data.Data_Transfer[1],0,TLF100.Write.Level_Base_Config.Audible,0,8)BTD(Port_Data.Data_Transfer[2],0,TLF100.Write.Level_Base_Config.Direction,0,8)BTD(Port_Data.Data_Transfer[3],0,TLF100.Write.Level_Base_Config.Percent_Width_of_Color_1,0,8)BTD(Port_Data.Data_Transfer[4],0,TLF100.Write.Level_Base_Config.Scroll_Bounce_Style,0,8)BTD(Port_Data.Data_Transfer[5],0,TLF100.Write.Level_Base_Config.Color_2_Intensity,0,8)BTD(Port_Data.Data_Transfer[6],0,TLF100.Write.Level_Base_Config.Color_2,0,8)BTD(Port_Data.Data_Transfer[7],0,TLF100.Write.Level_Base_Config.Pulse_Pattern,0,8)BTD(Port_Data.Data_Transfer[8],0,TLF100.Write.Level_Base_Config.Speed,0,8)BTD(Port_Data.Data_Transfer[9],0,TLF100.Write.Level_Base_Config.Color_1_Intensity,0,8)BTD(Port_Data.Data_Transfer[10],0,TLF100.Write.Level_Base_Config.Color_1,0,8)BTD(Port_Data.Data_Transfer[11],0,TLF100.Write.Level_Base_Config.Animation,0,8)OTU(Port_Data.Port_Read.[Port])OTL(Local_Control.6);
   34: NOP();
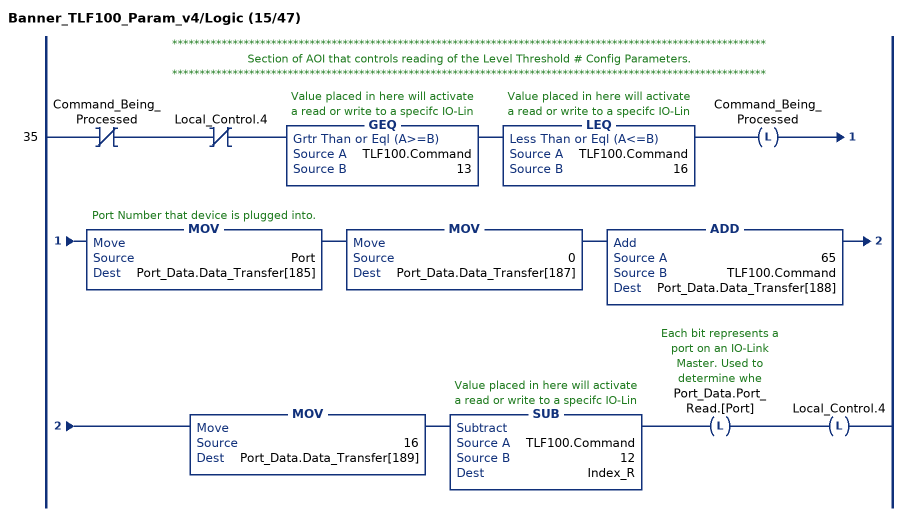
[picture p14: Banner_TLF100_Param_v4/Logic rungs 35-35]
   // ************************************************************************************************************
   // Section of AOI that controls reading of the Level Threshold # Config Parameters.
   // ************************************************************************************************************
   35: XIO(Command_Being_Processed)XIO(Local_Control.4)GEQ(TLF100.Command,13)LEQ(TLF100.Command,16)OTL(Command_Being_Processed)MOV(Port,Port_Data.Data_Transfer[185])MOV(0,Port_Data.Data_Transfer[187])ADD(65,TLF100.Command,Port_Data.Data_Transfer[188])MOV(16,Port_Data.Data_Transfer[189])SUB(TLF100.Command,12,Index_R)OTL(Port_Data.Port_Read.[Port])OTL(Local_Control.4);
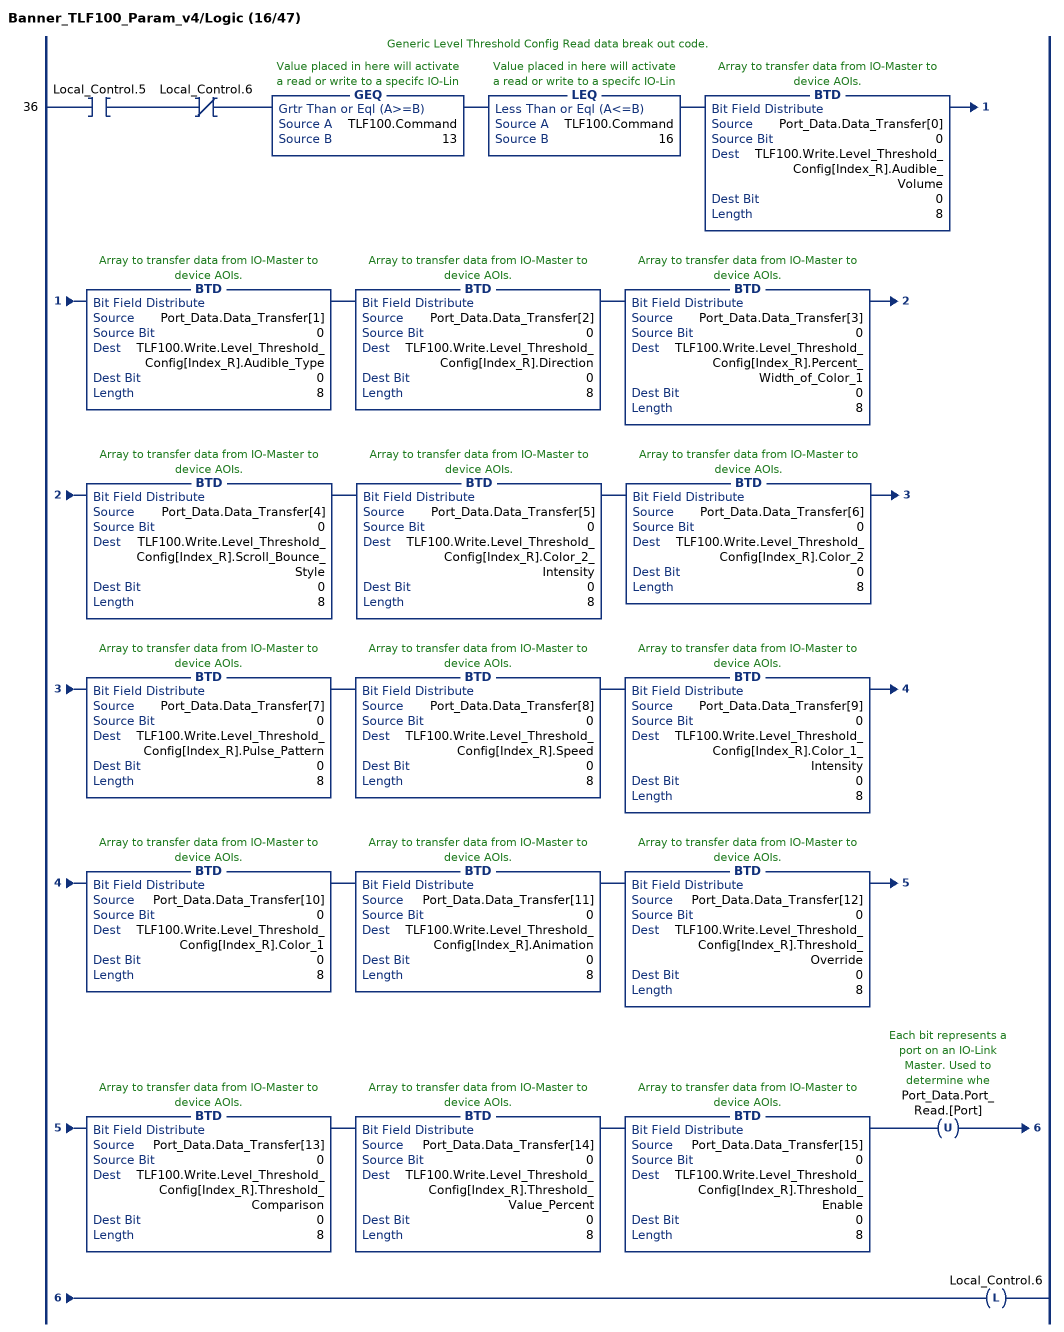
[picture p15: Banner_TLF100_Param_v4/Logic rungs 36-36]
   // Generic Level Threshold Config Read data break out code.
   36: XIC(Local_Control.5)XIO(Local_Control.6)GEQ(TLF100.Command,13)LEQ(TLF100.Command,16)BTD(Port_Data.Data_Transfer[0],0,TLF100.Write.Level_Threshold_Config[Index_R].Audible_Volume,0,8)BTD(Port_Data.Data_Transfer[1],0,TLF100.Write.Level_Threshold_Config[Index_R].Audible_Type,0,8)BTD(Port_Data.Data_Transfer[2],0,TLF100.Write.Level_Threshold_Config[Index_R].Direction,0,8)BTD(Port_Data.Data_Transfer[3],0,TLF100.Write.Level_Threshold_Config[Index_R].Percent_Width_of_Color_1,0,8)BTD(Port_Data.Data_Transfer[4],0,TLF100.Write.Level_Threshold_Config[Index_R].Scroll_Bounce_Style,0,8)BTD(Port_Data.Data_Transfer[5],0,TLF100.Write.Level_Threshold_Config[Index_R].Color_2_Intensity,0,8)BTD(Port_Data.Data_Transfer[6],0,TLF100.Write.Level_Threshold_Config[Index_R].Color_2,0,8)BTD(Port_Data.Data_Transfer[7],0,TLF100.Write.Level_Threshold_Config[Index_R].Pulse_Pattern,0,8)BTD(Port_Data.Data_Transfer[8],0,TLF100.Write.Level_Threshold_Config[Index_R].Speed,0,8)BTD(Port_Data.Data_Transfer[9],0,TLF100.Write.Level_Threshold_Config[Index_R].Color_1_Intensity,0,8)BTD(Port_Data.Data_Transfer[10],0,TLF100.Write.Level_Threshold_Config[Index_R].Color_1,0,8)BTD(Port_Data.Data_Transfer[11],0,TLF100.Write.Level_Threshold_Config[Index_R].Animation,0,8)BTD(Port_Data.Data_Transfer[12],0,TLF100.Write.Level_Threshold_Config[Index_R].Threshold_Override,0,8)BTD(Port_Data.Data_Transfer[13],0,TLF100.Write.Level_Threshold_Config[Index_R].Threshold_Comparison,0,8)BTD(Port_Data.Data_Transfer[14],0,TLF100.Write.Level_Threshold_Config[Index_R].Threshold_Value_Percent,0,8)BTD(Port_Data.Data_Transfer[15],0,TLF100.Write.Level_Threshold_Config[Index_R].Threshold_Enable,0,8)OTU(Port_Data.Port_Read.[Port])OTL(Local_Control.6);
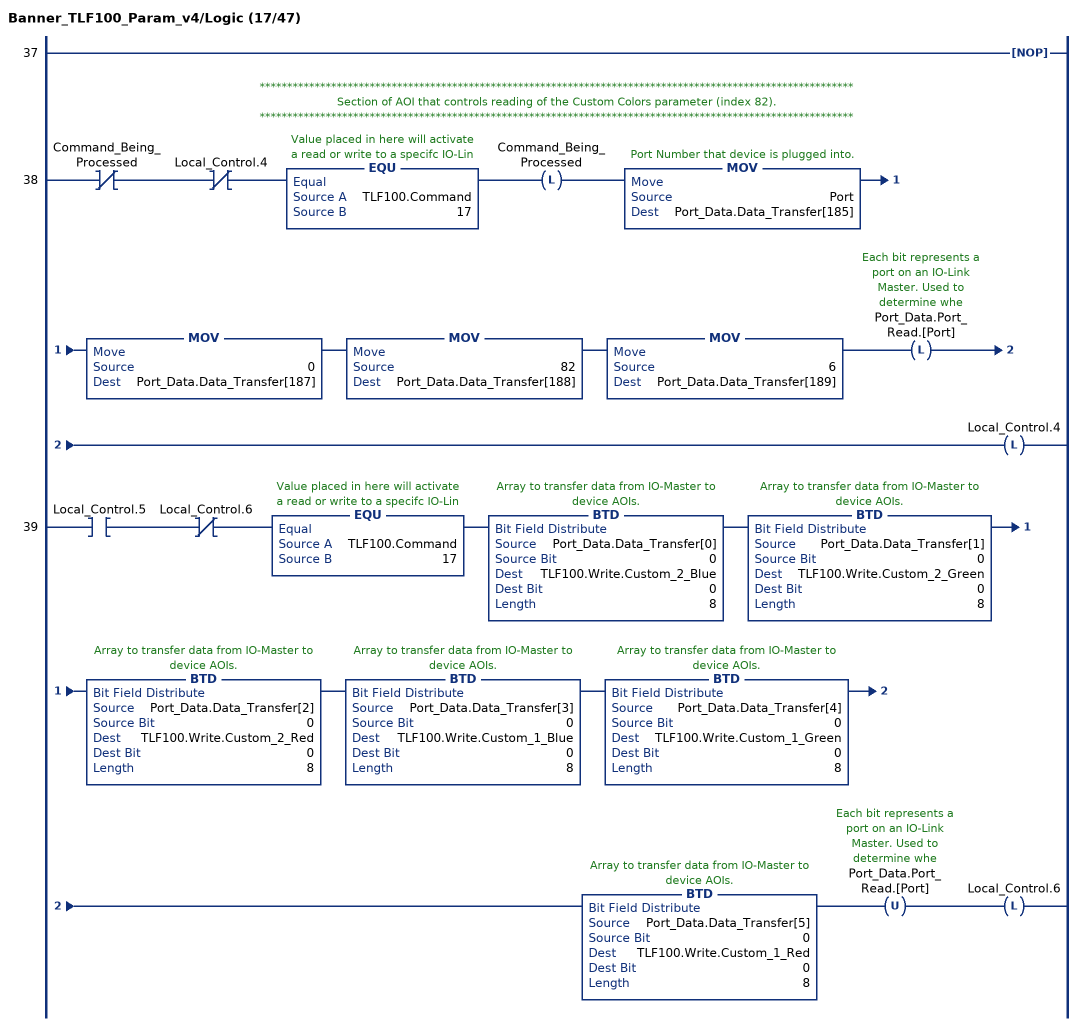
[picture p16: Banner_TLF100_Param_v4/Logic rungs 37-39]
   37: NOP();
   // ************************************************************************************************************
   // Section of AOI that controls reading of the Custom Colors parameter (index 82).
   // ************************************************************************************************************
   38: XIO(Command_Being_Processed)XIO(Local_Control.4)EQU(TLF100.Command,17)OTL(Command_Being_Processed)MOV(Port,Port_Data.Data_Transfer[185])MOV(0,Port_Data.Data_Transfer[187])MOV(82,Port_Data.Data_Transfer[188])MOV(6,Port_Data.Data_Transfer[189])OTL(Port_Data.Port_Read.[Port])OTL(Local_Control.4);
   39: XIC(Local_Control.5)XIO(Local_Control.6)EQU(TLF100.Command,17)BTD(Port_Data.Data_Transfer[0],0,TLF100.Write.Custom_2_Blue,0,8)BTD(Port_Data.Data_Transfer[1],0,TLF100.Write.Custom_2_Green,0,8)BTD(Port_Data.Data_Transfer[2],0,TLF100.Write.Custom_2_Red,0,8)BTD(Port_Data.Data_Transfer[3],0,TLF100.Write.Custom_1_Blue,0,8)BTD(Port_Data.Data_Transfer[4],0,TLF100.Write.Custom_1_Green,0,8)BTD(Port_Data.Data_Transfer[5],0,TLF100.Write.Custom_1_Red,0,8)OTU(Port_Data.Port_Read.[Port])OTL(Local_Control.6);
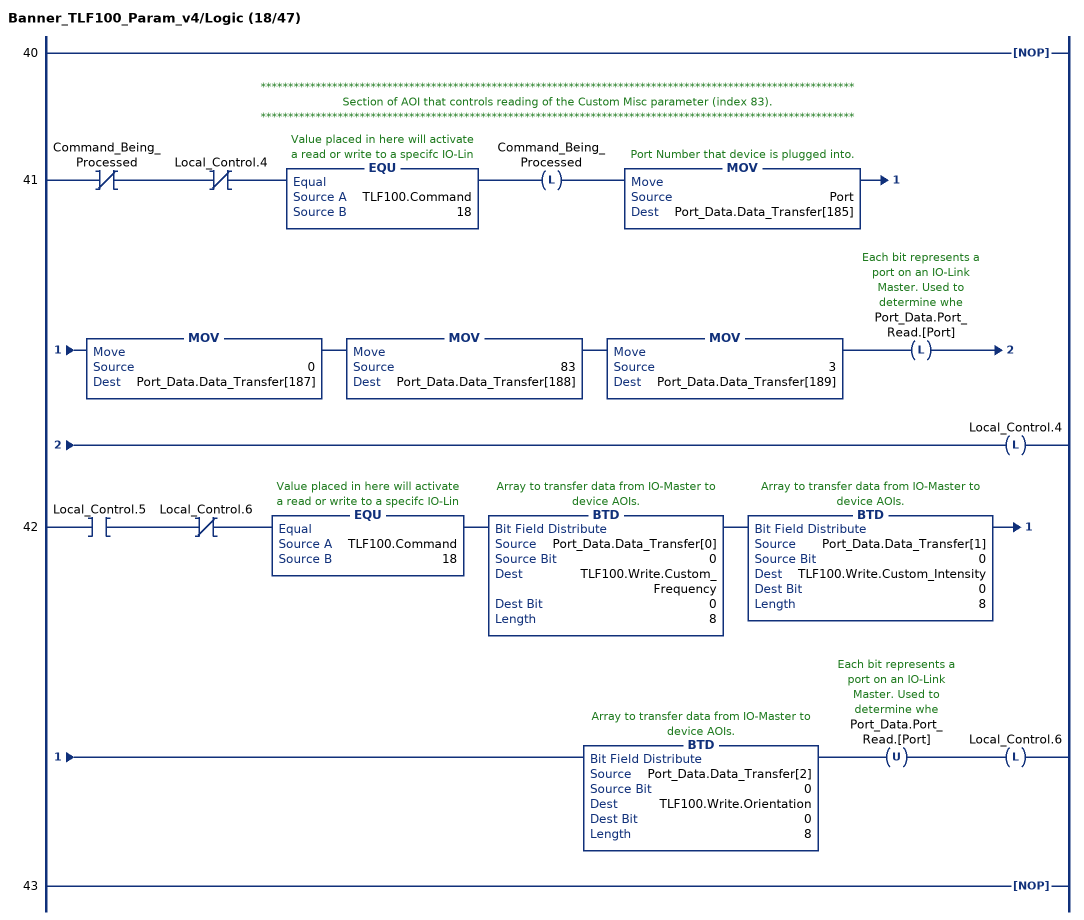
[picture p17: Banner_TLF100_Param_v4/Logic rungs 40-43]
   40: NOP();
   // ************************************************************************************************************
   // Section of AOI that controls reading of the Custom Misc parameter (index 83).
   // ************************************************************************************************************
   41: XIO(Command_Being_Processed)XIO(Local_Control.4)EQU(TLF100.Command,18)OTL(Command_Being_Processed)MOV(Port,Port_Data.Data_Transfer[185])MOV(0,Port_Data.Data_Transfer[187])MOV(83,Port_Data.Data_Transfer[188])MOV(3,Port_Data.Data_Transfer[189])OTL(Port_Data.Port_Read.[Port])OTL(Local_Control.4);
   42: XIC(Local_Control.5)XIO(Local_Control.6)EQU(TLF100.Command,18)BTD(Port_Data.Data_Transfer[0],0,TLF100.Write.Custom_Frequency,0,8)BTD(Port_Data.Data_Transfer[1],0,TLF100.Write.Custom_Intensity,0,8)BTD(Port_Data.Data_Transfer[2],0,TLF100.Write.Orientation,0,8)OTU(Port_Data.Port_Read.[Port])OTL(Local_Control.6);
   43: NOP();
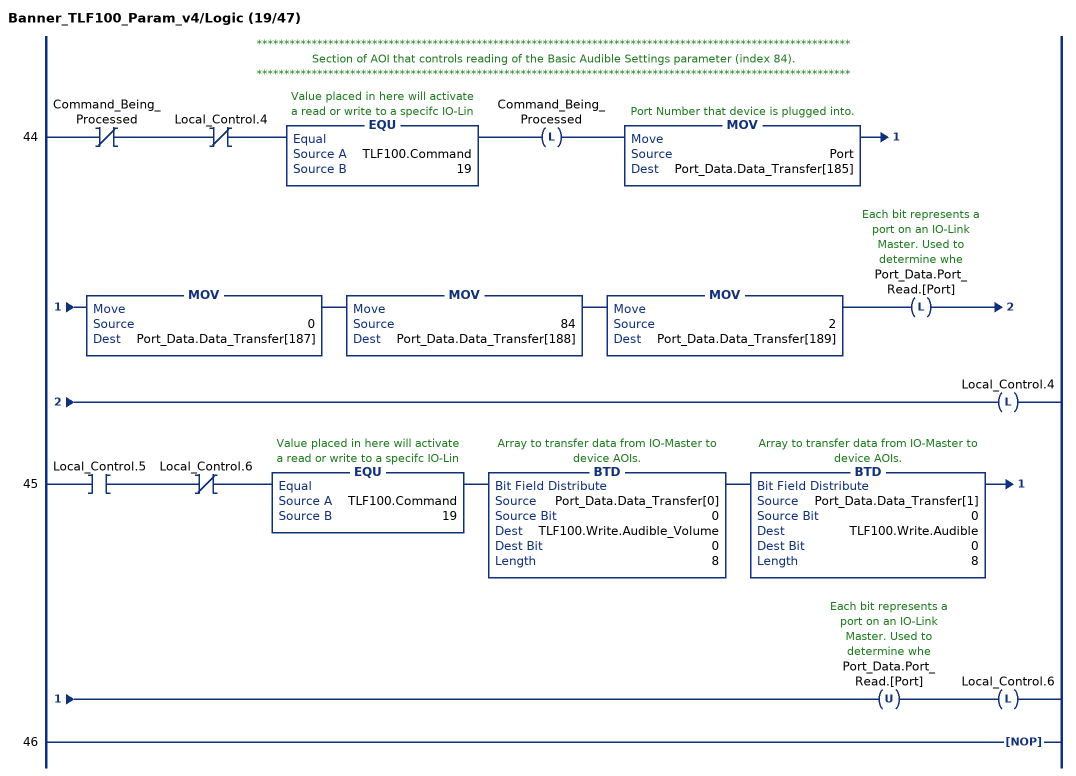
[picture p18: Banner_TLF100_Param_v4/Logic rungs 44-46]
   // ************************************************************************************************************
   // Section of AOI that controls reading of the Basic Audible Settings parameter (index 84).
   // ************************************************************************************************************
   44: XIO(Command_Being_Processed)XIO(Local_Control.4)EQU(TLF100.Command,19)OTL(Command_Being_Processed)MOV(Port,Port_Data.Data_Transfer[185])MOV(0,Port_Data.Data_Transfer[187])MOV(84,Port_Data.Data_Transfer[188])MOV(2,Port_Data.Data_Transfer[189])OTL(Port_Data.Port_Read.[Port])OTL(Local_Control.4);
   45: XIC(Local_Control.5)XIO(Local_Control.6)EQU(TLF100.Command,19)BTD(Port_Data.Data_Transfer[0],0,TLF100.Write.Audible_Volume,0,8)BTD(Port_Data.Data_Transfer[1],0,TLF100.Write.Audible,0,8)OTU(Port_Data.Port_Read.[Port])OTL(Local_Control.6);
   46: NOP();
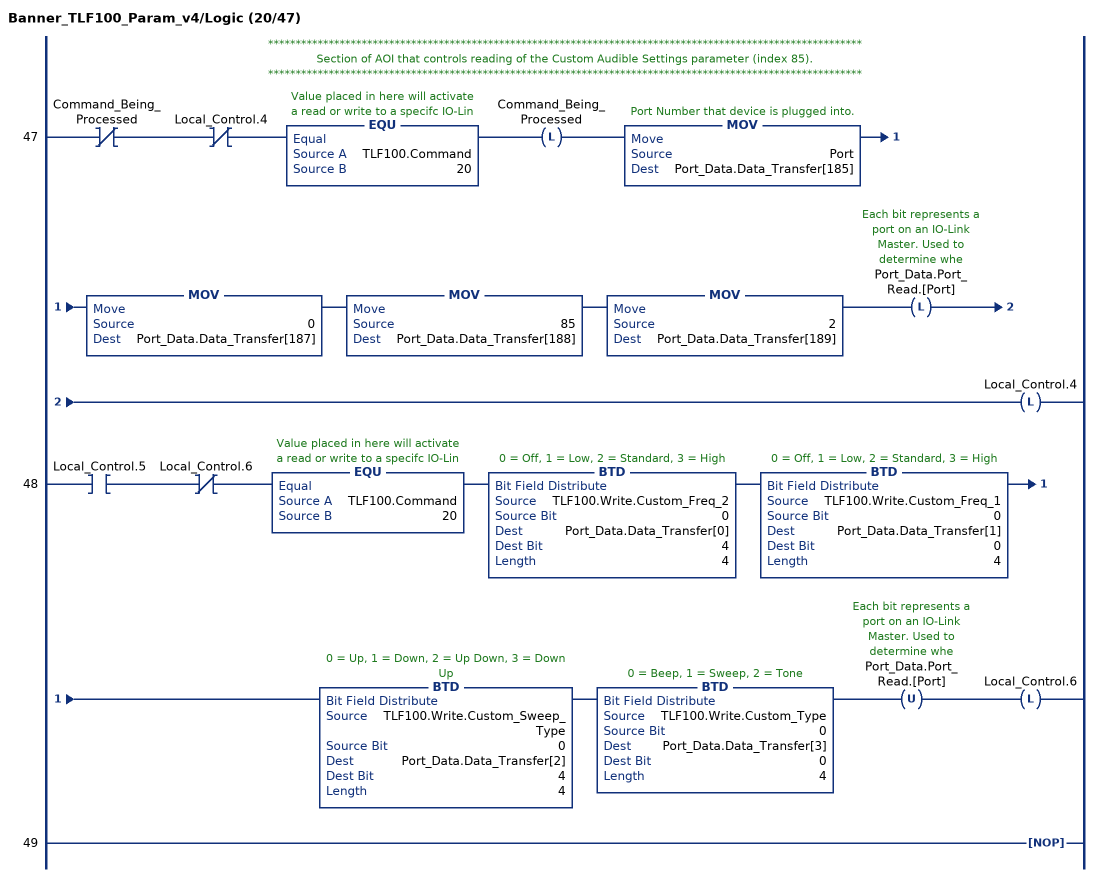
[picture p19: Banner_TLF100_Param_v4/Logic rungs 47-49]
   // ************************************************************************************************************
   // Section of AOI that controls reading of the Custom Audible Settings parameter (index 85).
   // ************************************************************************************************************
   47: XIO(Command_Being_Processed)XIO(Local_Control.4)EQU(TLF100.Command,20)OTL(Command_Being_Processed)MOV(Port,Port_Data.Data_Transfer[185])MOV(0,Port_Data.Data_Transfer[187])MOV(85,Port_Data.Data_Transfer[188])MOV(2,Port_Data.Data_Transfer[189])OTL(Port_Data.Port_Read.[Port])OTL(Local_Control.4);
   48: XIC(Local_Control.5)XIO(Local_Control.6)EQU(TLF100.Command,20)BTD(TLF100.Write.Custom_Freq_2,0,Port_Data.Data_Transfer[0],4,4)BTD(TLF100.Write.Custom_Freq_1,0,Port_Data.Data_Transfer[1],0,4)BTD(TLF100.Write.Custom_Sweep_Type,0,Port_Data.Data_Transfer[2],4,4)BTD(TLF100.Write.Custom_Type,0,Port_Data.Data_Transfer[3],0,4)OTU(Port_Data.Port_Read.[Port])OTL(Local_Control.6);
   49: NOP();
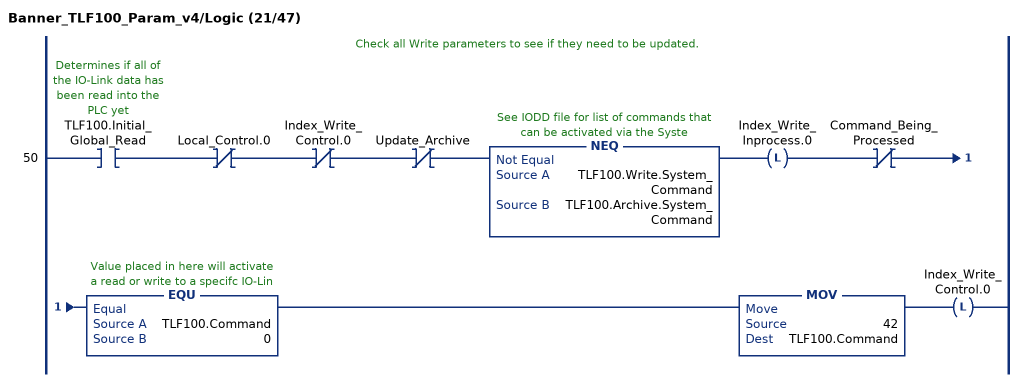
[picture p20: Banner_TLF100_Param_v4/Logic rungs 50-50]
   // Check all Write parameters to see if they need to be updated.
   50: XIC(TLF100.Initial_Global_Read)XIO(Local_Control.0)XIO(Index_Write_Control.0)XIO(Update_Archive)NEQ(TLF100.Write.System_Command,TLF100.Archive.System_Command)OTL(Index_Write_Inprocess.0)XIO(Command_Being_Processed)EQU(TLF100.Command,0)MOV(42,TLF100.Command)OTL(Index_Write_Control.0);
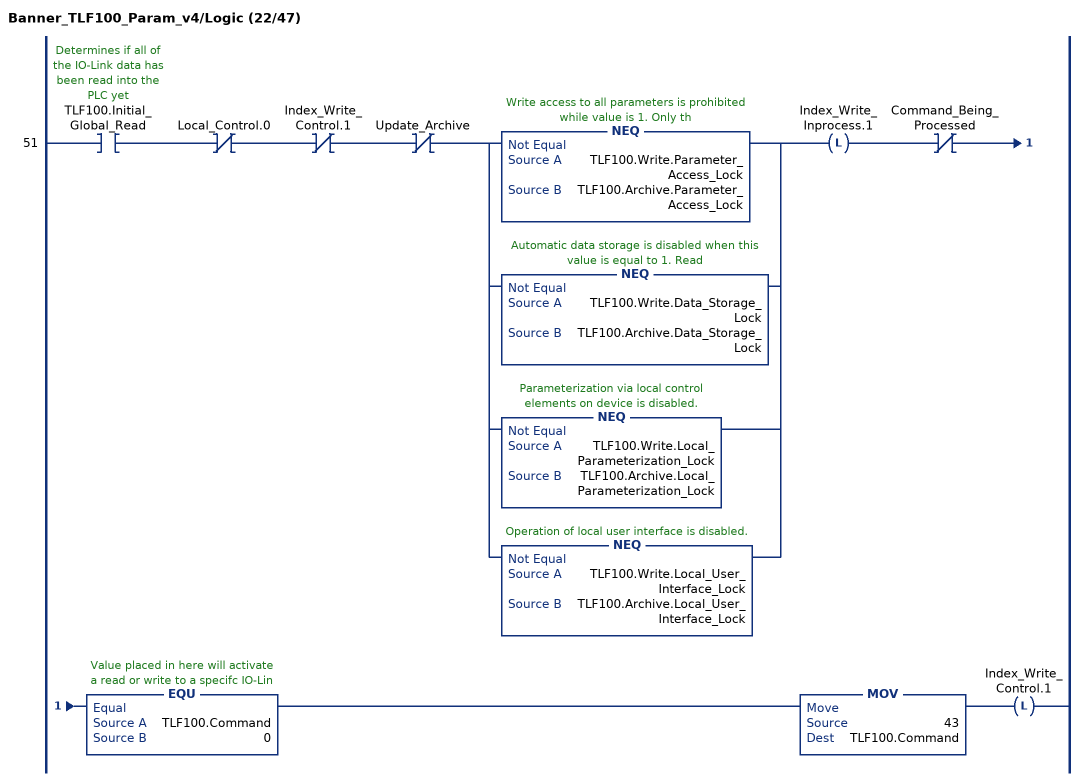
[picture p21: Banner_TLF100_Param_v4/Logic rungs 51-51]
   51: XIC(TLF100.Initial_Global_Read)XIO(Local_Control.0)XIO(Index_Write_Control.1)XIO(Update_Archive)[NEQ(TLF100.Write.Parameter_Access_Lock,TLF100.Archive.Parameter_Access_Lock) ,NEQ(TLF100.Write.Data_Storage_Lock,TLF100.Archive.Data_Storage_Lock) ,NEQ(TLF100.Write.Local_Parameterization_Lock,TLF100.Archive.Local_Parameterization_Lock) ,NEQ(TLF100.Write.Local_User_Interface_Lock,TLF100.Archive.Local_User_Interface_Lock) ]OTL(Index_Write_Inprocess.1)XIO(Command_Being_Processed)EQU(TLF100.Command,0)MOV(43,TLF100.Command)OTL(Index_Write_Control.1);
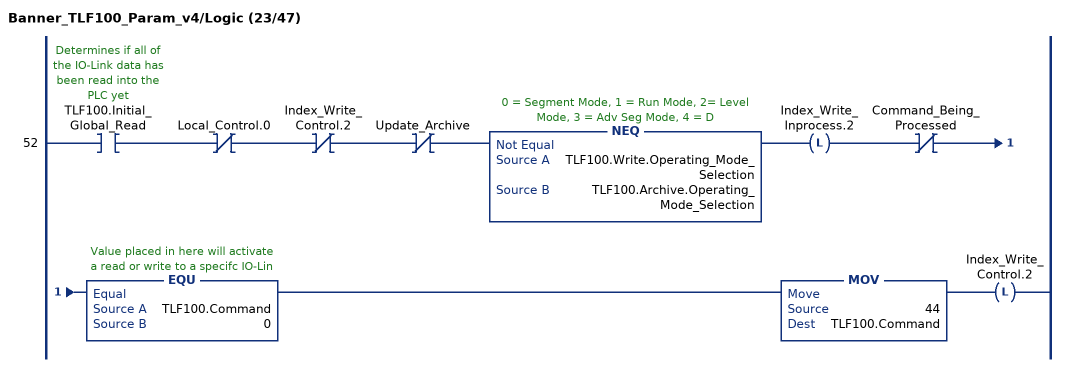
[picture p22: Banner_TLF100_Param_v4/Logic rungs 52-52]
   52: XIC(TLF100.Initial_Global_Read)XIO(Local_Control.0)XIO(Index_Write_Control.2)XIO(Update_Archive)NEQ(TLF100.Write.Operating_Mode_Selection,TLF100.Archive.Operating_Mode_Selection)OTL(Index_Write_Inprocess.2)XIO(Command_Being_Processed)EQU(TLF100.Command,0)MOV(44,TLF100.Command)OTL(Index_Write_Control.2);
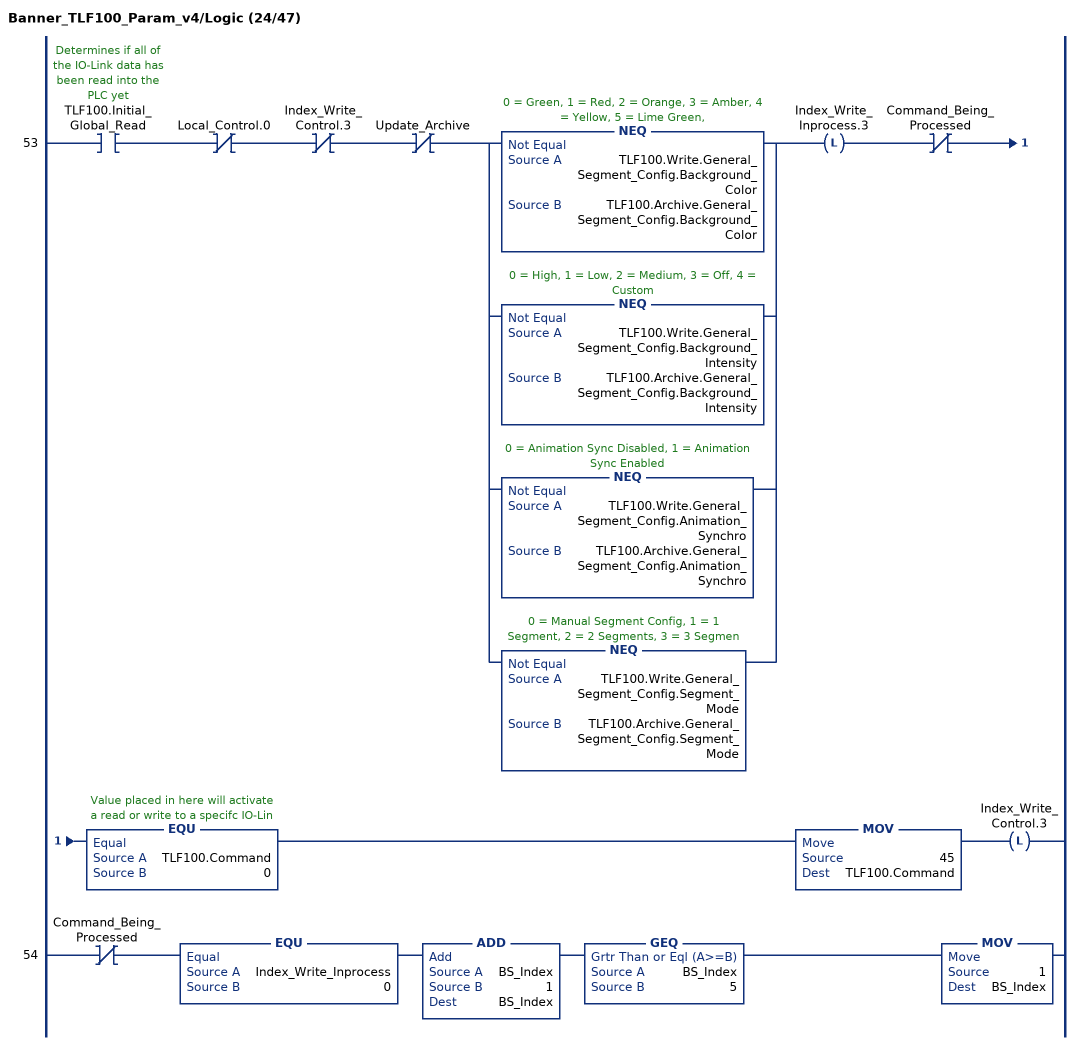
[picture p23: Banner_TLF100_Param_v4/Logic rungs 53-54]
   53: XIC(TLF100.Initial_Global_Read)XIO(Local_Control.0)XIO(Index_Write_Control.3)XIO(Update_Archive)[NEQ(TLF100.Write.General_Segment_Config.Background_Color,TLF100.Archive.General_Segment_Config.Background_Color) ,NEQ(TLF100.Write.General_Segment_Config.Background_Intensity,TLF100.Archive.General_Segment_Config.Background_Intensity) ,NEQ(TLF100.Write.General_Segment_Config.Animation_Synchro,TLF100.Archive.General_Segment_Config.Animation_Synchro) ,NEQ(TLF100.Write.General_Segment_Config.Segment_Mode,TLF100.Archive.General_Segment_Config.Segment_Mode) ]OTL(Index_Write_Inprocess.3)XIO(Command_Being_Processed)EQU(TLF100.Command,0)MOV(45,TLF100.Command)OTL(Index_Write_Control.3);
   54: XIO(Command_Being_Processed)EQU(Index_Write_Inprocess,0)ADD(BS_Index,1,BS_Index)GEQ(BS_Index,5)MOV(1,BS_Index);
